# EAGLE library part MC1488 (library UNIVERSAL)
MC1488 RS232 quad line driver. Supply +12V/-12v
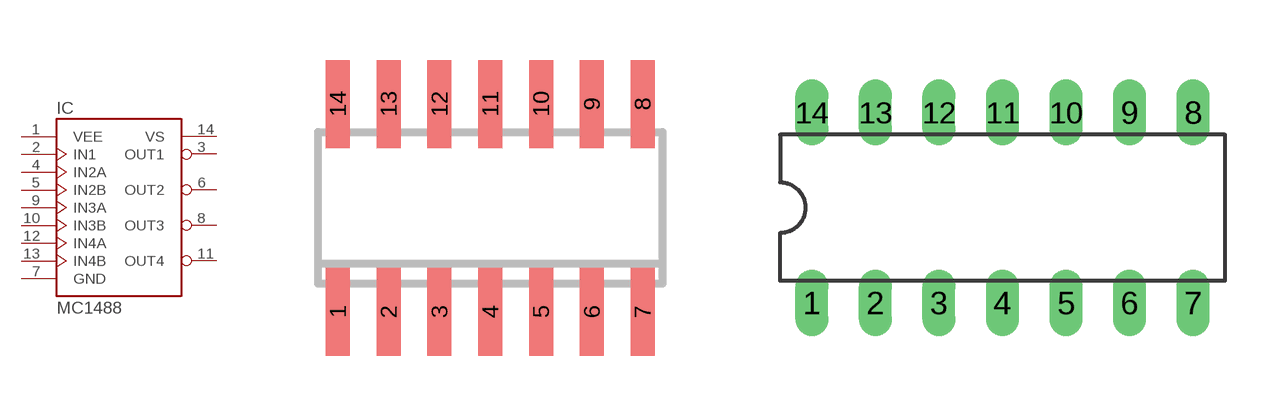
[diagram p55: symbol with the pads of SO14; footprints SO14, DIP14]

Designator prefix IC

## MC1488D (IC: mc1488)  [SO14]
1  VEE  pwr
2  IN1  in
3  OUT1  out
4  IN2A  in
5  IN2B  in
6  OUT2  out
7  GND  sup
8  OUT3  out
9  IN3A  in
10  IN3B  in
11  OUT4  out
12  IN4A  in
13  IN4B  in
14  VS  pwr

## MC1488  [DIP14]
Pads as for SO14

## Footprint SO14 (pad centres in mm)
smd 0.6 x 2.2: 1 -3.81,-2.6; 2 -2.54,-2.6; 3 -1.27,-2.6; 4 0,-2.6; 5 1.27,-2.6; 6 2.54,-2.6; 7 3.81,-2.6; 8 3.81,2.6; 9 2.54,2.6; 10 1.27,2.6; 11 0,2.6; 12 -1.27,2.6; 13 -2.54,2.6; 14 -3.81,2.6

## Footprint DIP14 (pad centres in mm)
drill 0.813 long: 1 0,0; 2 2.54,0; 3 5.08,0; 4 7.62,0; 5 10.16,0; 6 12.7,0; 7 15.24,0; 8 15.24,7.62; 9 12.7,7.62; 10 10.16,7.62; 11 7.62,7.62; 12 5.08,7.62; 13 2.54,7.62; 14 0,7.62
